TYPE E_IEC870_5_101MState :
(
	e101MState_Init := 0,
	e101MState_CycleStart,
	
	e101MState_TestAct,
	e101MState_TestCon,
	
	e101MState_ClockAct,
	e101MState_ClockCon,
	
	e101MState_GeninAct,
	e101MState_GeninCon,
	e101MState_GeninTerm,
	
	e101MState_Coro,
	e101MState_CoroFrzRstAct,
	e101MState_CoroFrzRstCon,
	e101MState_CoroReadAct,
	e101MState_CoroReadCon,
	e101MState_CoroReadTerm,
	
	e101MState_CmdAct,
	e101MState_CmdCon,
	e101MState_CmdTerm,
	e101MState_CycleEnd
);
END_TYPE
